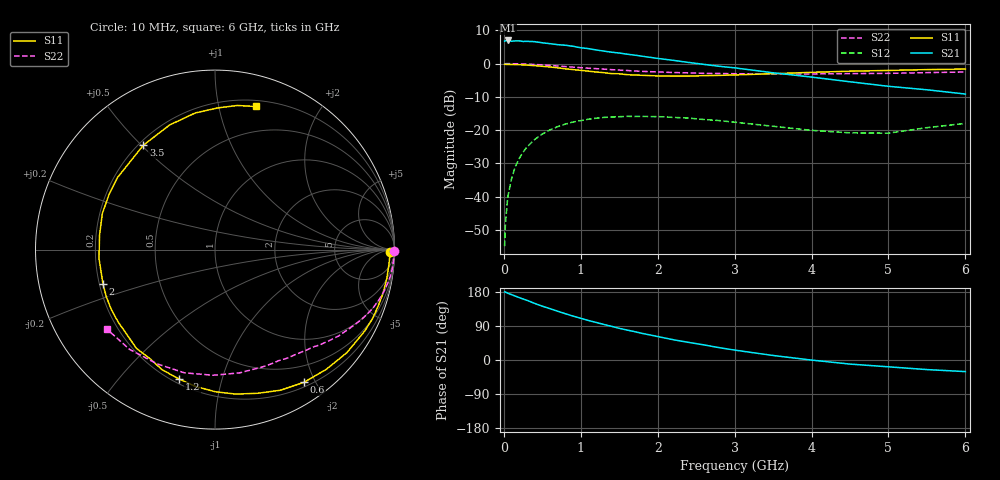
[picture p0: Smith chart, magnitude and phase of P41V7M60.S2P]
! SIEMENS Small Signal Semiconductors
! BFP182
! Si NPN RF Bipolar Junction Transistor in SOT143
! VCE = 1.75 V  IC = 0.6 mA
! Common Emitter S-Parameters:  March  1996
# GHz  S  MA  R  50
!  f  S11  S21  S12  S22
! GHz  MAG  ANG  MAG  ANG  MAG  ANG  MAG  ANG
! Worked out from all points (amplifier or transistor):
!   36 points, 10 MHz to 6 GHz, reference 50 ohm
!   highest |S21| = 7.0 dB at 50 MHz (marker M1)
!   |S21| within 3 dB of that: start of sweep to 1.244 GHz
!   unconditionally stable (mu >= 1): 2.863 GHz to end of sweep
!   at 250 MHz: K = 0.09, MSG = 16.6 dB, |S12| = -26.6 dB
!   at 1.4 GHz: K = 0.51, MSG = 9.7 dB, |S12| = -16.1 dB
!   at 6 GHz: K = 1.20, MAG = 1.7 dB, |S12| = -18.0 dB
!   S11 on the Smith chart (normalised r, x): 10 MHz: 60, -41; 600 MHz: 0.26, -1.85; 1.2 GHz: 0.22, -0.73; 2 GHz: 0.21, -0.14; 3.5 GHz: 0.22, +0.51; 6 GHz: 0.25, +1.29
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0.01  0.9776 -0.9  2.174 179.7  0.0018 87.5  0.9995 -0.3
0.02  0.9745 -2.0  2.206 179.3  0.0038 89.0  0.9962 -0.7
0.05  0.9726 -5.0  2.229 176.3  0.0097 89.5  0.9997 -1.8
0.1  0.9707 -9.5  2.173 172.5  0.0187 83.1  0.9959 -3.6
0.15  0.9674 -14.5  2.197 168.6  0.0283 80.2  0.9944 -5.4
0.25  0.9582 -23.7  2.154 161.0  0.0467 74.7  0.9873 -8.9
0.4  0.9324 -38.0  2.139 149.3  0.0721 65.4  0.97 -13.9
0.6  0.8903 -56.1  1.995 135.5  0.1009 54.0  0.9392 -20.1
0.8  0.8353 -73.4  1.889 122.1  0.1231 43.8  0.9034 -25.6
1.1  0.7698 -98.2  1.68 104.2  0.1459 30.3  0.853 -32.7
1.2  0.748 -105.6  1.605 99.1  0.151 26.1  0.84 -35.0
1.5  0.7032 -128.6  1.444 83.6  0.159 15.8  0.7988 -40.7
1.8  0.6674 -149.9  1.29 70.1  0.1606 7.5  0.765 -45.9
2  0.653 -162.9  1.197 61.9  0.1597 2.4  0.7495 -49.2
2.2  0.6481 -175.6  1.121 53.6  0.1555 -2.3  0.7354 -52.9
2.6  0.6592 162.2  0.974 39.9  0.1444 -9.2  0.7133 -60.1
3  0.6754 143.5  0.864 26.2  0.1315 -14.7  0.7049 -68.1
3.5  0.7054 124.5  0.728 11.9  0.1143 -16.9  0.7004 -78.8
4.5  0.7692 98.2  0.533 -10.8  0.091 -6.8  0.7074 -103.9
5  0.7895 88.9  0.456 -18.0  0.09 6.4  0.7137 -117.0
5.5  0.8125 81.2  0.404 -25.3  0.1089 12.1  0.7319 -130.6
6  0.829 74.1  0.349 -30.6  0.1264 13.0  0.7474 -143.6
